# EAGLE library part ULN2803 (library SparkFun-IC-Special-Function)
Darlington Driver(IC-07959, low stock) ULN2803 Darlington array. 500mA max per channel, 8-channel package. Spark Fun Electronics SKU : COM-00312
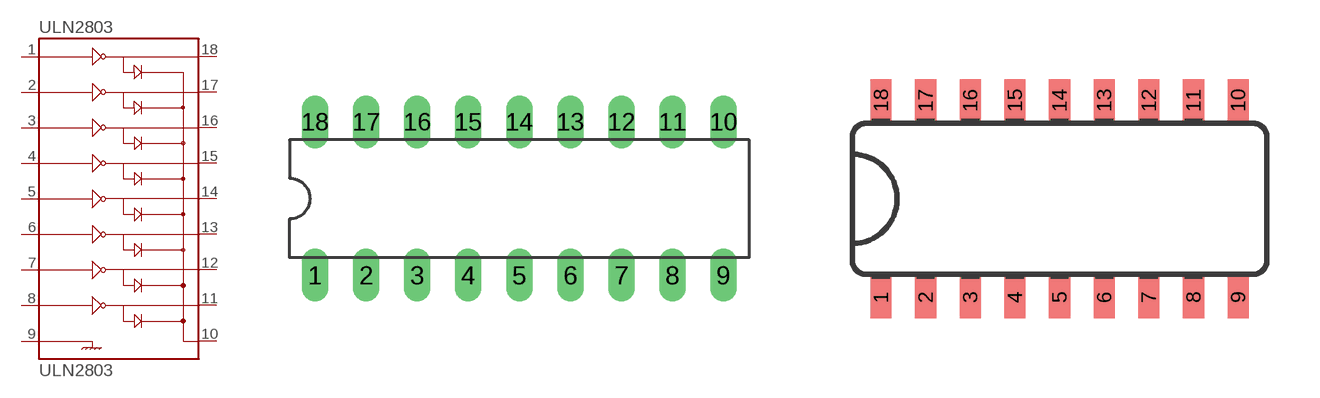
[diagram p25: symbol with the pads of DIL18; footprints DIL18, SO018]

Designator prefix ULN2803

## ULN2803DIP  [DIL18]
1  1
2  2
3  3
4  4
5  5
6  6
7  7
8  8
9  9
10  10
11  11
12  12
13  13
14  14
15  15
16  16
17  17
18  18

## ULN2803SOIC  [SO018]
Pads as for DIL18

## ULN2803SOICW  [SO18L]
Pads as for DIL18

## Footprint DIL18 (pad centres in mm)
Dual In Line Package - 18 Pin Specifications: Pin count: 18 Example device(s): LM391
drill 0.813 long: 1 -10.16,-3.81; 2 -7.62,-3.81; 3 -5.08,-3.81; 4 -2.54,-3.81; 5 0,-3.81; 6 2.54,-3.81; 7 5.08,-3.81; 8 7.62,-3.81; 9 10.16,-3.81; 10 10.16,3.81; 11 7.62,3.81; 12 5.08,3.81; 13 2.54,3.81; 14 0,3.81; 15 -2.54,3.81; 16 -5.08,3.81; 17 -7.62,3.81; 18 -10.16,3.81

## Footprint SO018 (pad centres in mm)
smd 0.6 x 1.2: 1 -5.08,-2.8; 2 -3.81,-2.8; 3 -2.54,-2.8; 4 -1.27,-2.8; 5 0,-2.8; 6 1.27,-2.8; 7 2.54,-2.8; 8 3.81,-2.8; 9 5.08,-2.8; 10 5.08,2.8; 11 3.81,2.8; 12 2.54,2.8; 13 1.27,2.8; 14 0,2.8; 15 -1.27,2.8; 16 -2.54,2.8; 17 -3.81,2.8; 18 -5.08,2.8

## Footprint SO18L (pad centres in mm)
smd 0.66 x 2.032: 1 -0.635,-4.902; 2 0.635,-4.902; 3 1.905,-4.902; 4 3.175,-4.902; 5 4.445,-4.902; 6 5.715,-4.902; 7 6.985,-4.902; 8 8.255,-4.902; 9 9.525,-4.902; 10 9.525,4.902; 11 8.255,4.902; 12 6.985,4.902; 13 5.715,4.902; 14 4.445,4.902; 15 3.175,4.902; 16 1.905,4.902; 17 0.635,4.902; 18 -0.635,4.902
